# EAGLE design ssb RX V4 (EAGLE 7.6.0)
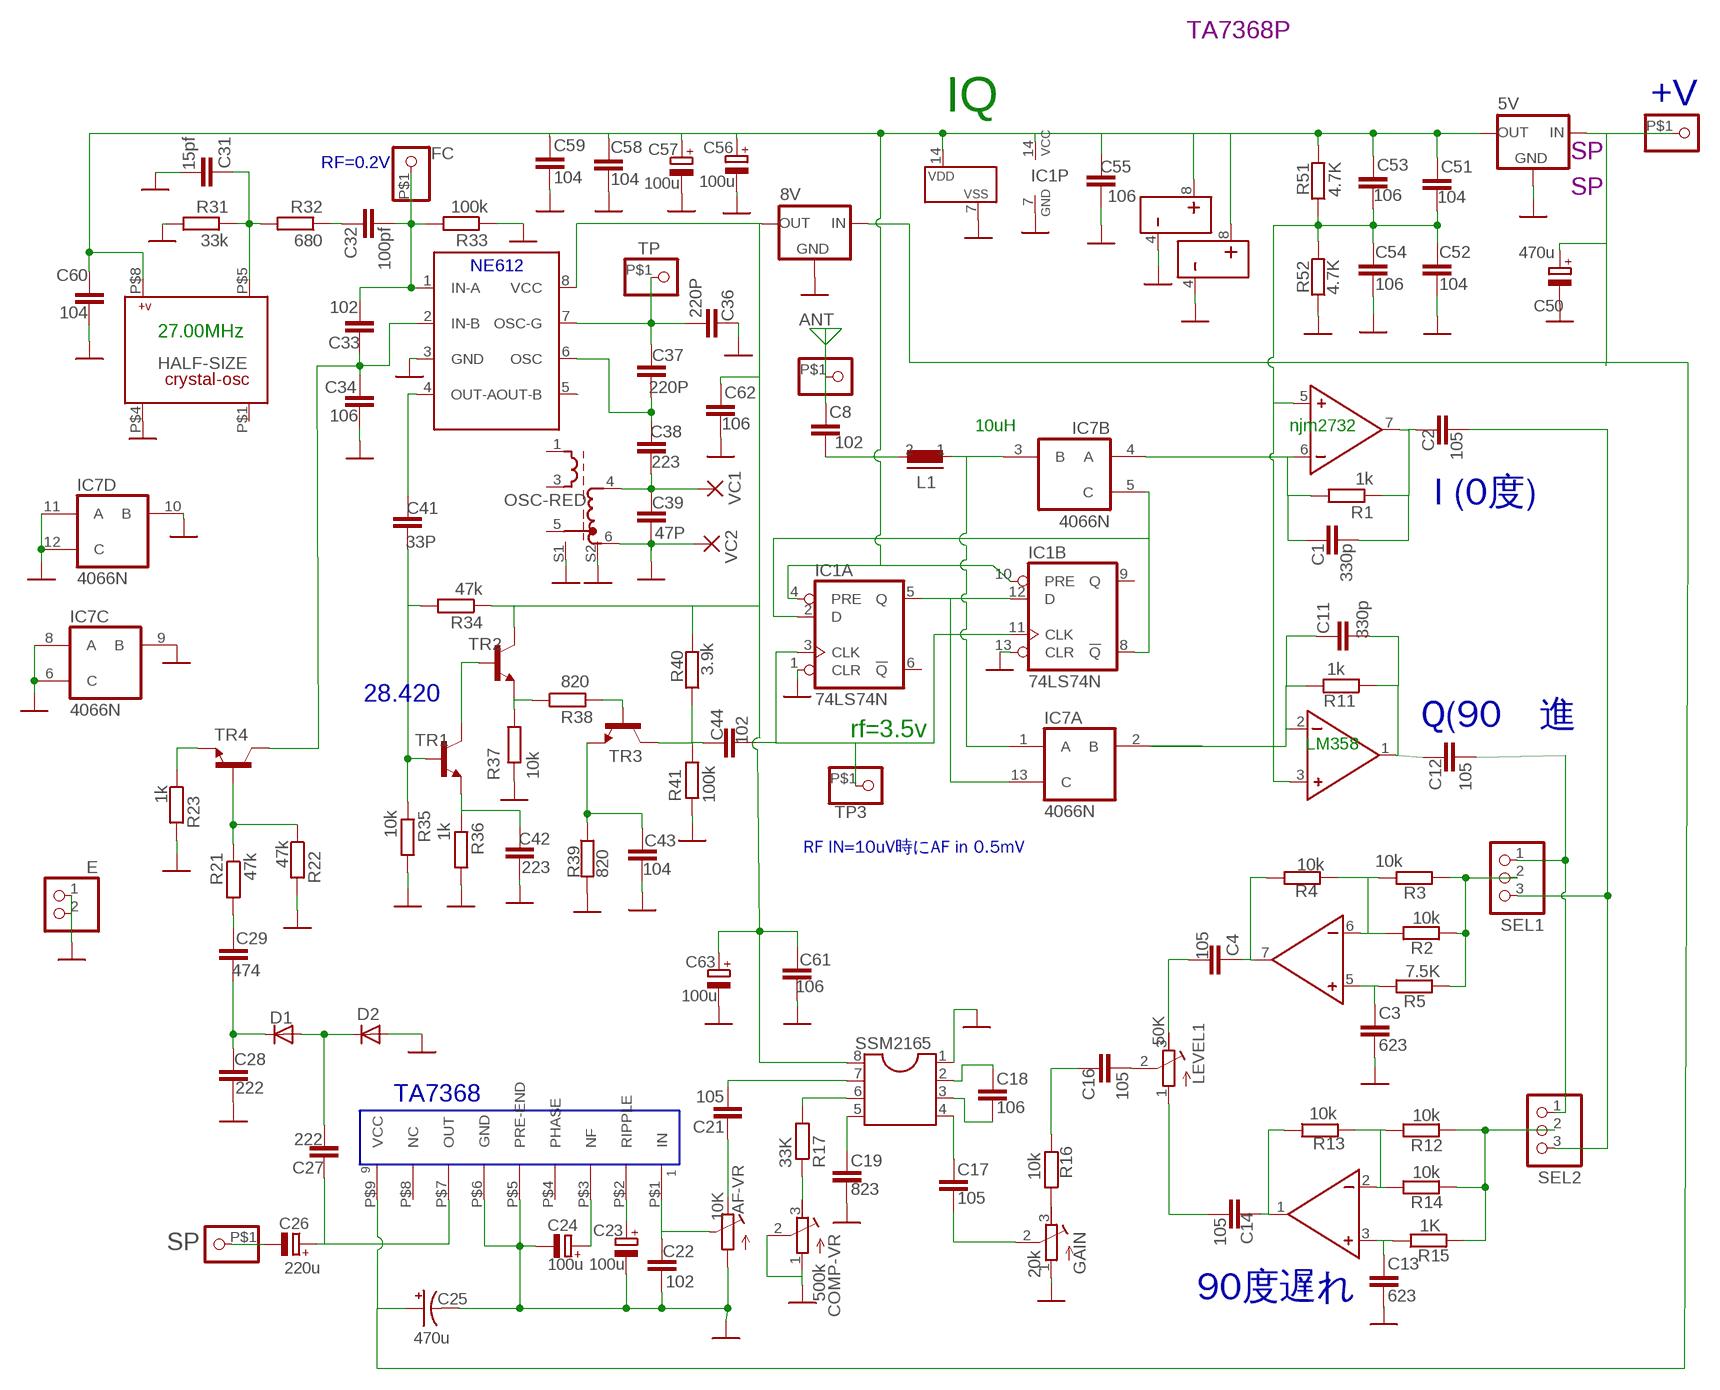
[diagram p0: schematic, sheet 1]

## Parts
5V  78MXX  [78MXX]
8V  78MXX  [78MXX]
+V  PINHD-1X1  [1X01]
AF-VR  10K  SINGLE-VR  [SINGLE-VR]
ANT  PINHD-1X1  [1X01]
C1  330p  C-EU050-024X044  [C050-024X044]
C2  105  C-EU050-024X044  [C050-024X044]
C3  623  C-EU050-024X044  [C050-024X044]
C4  105  C-EU050-024X044  [C050-024X044]
C8  102  C-EU050-024X044  [C050-024X044]
C11  330p  C-EU050-024X044  [C050-024X044]
C12  105  C-EU050-024X044  [C050-024X044]
C13  623  C-EU050-024X044  [C050-024X044]
C14  105  C-EU050-024X044  [C050-024X044]
C16  105  C-EU050-024X044  [C050-024X044]
C17  105  C-EU050-024X044  [C050-024X044]
C18  106  C-EU050-024X044  [C050-024X044]
C19  823  C-EU050-024X044  [C050-024X044]
C21  105  C-EU050-024X044  [C050-024X044]
C22  102  C-EU050-024X044  [C050-024X044]
C23  100u  CPOL-EUE2.5-6  [E2,5-6]
C24  100u  CPOL-EUE2.5-6  [E2,5-6]
C25  470u  CPOL-USE3.5-8  [E3,5-8]
C26  220u  CPOL-EUE2.5-6  [E2,5-6]
C27  222  C-EU050-024X044  [C050-024X044]
C28  222  C-EU050-024X044  [C050-024X044]
C29  474  C-EU050-024X044  [C050-024X044]
C31  15pf  C-EU050-024X044  [C050-024X044]
C32  100pf  C-EU050-024X044  [C050-024X044]
C33  102  C-EU050-024X044  [C050-024X044]
C34  106  C-EU050-024X044  [C050-024X044]
C36  220P  C-EU050-024X044  [C050-024X044]
C37  220P  C-EU050-024X044  [C050-024X044]
C38  223  C-EU050-024X044  [C050-024X044]
C39  47P  C-EU050-024X044  [C050-024X044]
C41  33P  C-EU050-024X044  [C050-024X044]
C42  223  C-EU050-024X044  [C050-024X044]
C43  104  C-EU050-024X044  [C050-024X044]
C44  102  C-EU050-024X044  [C050-024X044]
C50  470u  CPOL-EUE2.5-7  [E2,5-7]
C51  104  C-EU050-024X044  [C050-024X044]
C52  104  C-EU050-024X044  [C050-024X044]
C53  106  C-EU050-024X044  [C050-024X044]
C54  106  C-EU050-024X044  [C050-024X044]
C55  106  C-EU050-024X044  [C050-024X044]
C56  100u  CPOL-EUE2.5-6  [E2,5-6]
C57  100u  CPOL-EUE2.5-6  [E2,5-6]
C58  104  C-EU050-024X044  [C050-024X044]
C59  104  C-EU050-024X044  [C050-024X044]
C60  104  C-EU050-024X044  [C050-024X044]
C61  106  C-EU050-024X044  [C050-024X044]
C62  106  C-EU050-024X044  [C050-024X044]
C63  100u  CPOL-EUE2.5-6  [E2,5-6]
COMP-VR  500k  R-TRIMM3296W  [RTRIM3296W]
D1  DIODE-D-5  [D-5]
D2  DIODE-D-5  [D-5]
E  PINHD-1X2  [1X02]
FC  FC  PINHD-1X1  [1X01]
GAIN  20k  R-TRIMM3296W  [RTRIM3296W]
HALF-SIZE  X-OSC  [X-OSC]
IC1  74LS74N  [DIL14]
IC3  NE612  [NE612]
IC4  4558  [DIL08]
IC5  4558  [DIL08]
IC7  4066N  [DIL14]
JP1  SEL1  PINHD-1X3  [1X03]
JP3  SEL2  PINHD-1X3  [1X03]
L1  MCC10  [MCC10]
LEVEL1  50K  R-TRIMM3296W  [RTRIM3296W]
R1  1k  R-EU_0204/5  [0204/5]
R2  10k  R-EU_0204/5  [0204/5]
R3  10k  R-EU_0204/5  [0204/5]
R4  10k  R-EU_0204/5  [0204/5]
R5  7.5K  R-EU_0204/5  [0204/5]
R11  1k  R-EU_0204/5  [0204/5]
R12  10k  R-EU_0204/7  [0204/7]
R13  10k  R-EU_0204/5  [0204/5]
R14  10k  R-EU_0204/7  [0204/7]
R15  1K  R-EU_0204/5  [0204/5]
R16  10k  R-EU_0204/5  [0204/5]
R17  33K  R-EU_0204/5  [0204/5]
R21  47k  R-EU_0204/5  [0204/5]
R22  47k  R-EU_0204/5  [0204/5]
R23  1k  R-EU_0204/5  [0204/5]
R31  33k  R-EU_0204/5  [0204/5]
R32  680  R-EU_0204/5  [0204/5]
R33  100k  R-EU_0204/5  [0204/5]
R34  47k  R-EU_0204/5  [0204/5]
R35  10k  R-EU_0204/5  [0204/5]
R36  1k  R-EU_0204/5  [0204/5]
R37  10k  R-EU_0204/7  [0204/7]
R38  820  R-EU_0204/5  [0204/5]
R39  820  R-EU_0204/5  [0204/5]
R40  3.9k  R-EU_0204/5  [0204/5]
R41  100k  R-EU_0204/5  [0204/5]
R51  4.7K  R-EU_0204/5  [0204/5]
R52  4.7K  R-EU_0204/5  [0204/5]
SP  PINHD-1X1  [1X01]
SSM2165  LM386  [DIL08]
TA7368  TA7368P  [TA7368P]
TP  PINHD-1X1  [1X01]
TP3  PINHD-1X1  [1X01]
TR1  2SC1815L  [TO92-1815]
TR2  2SC1815L  [TO92-1815]
TR3  2SC1815L  [TO92-1815]
TR4  2SC1815L  [TO92-1815]
U$3  OSC-RED  [OSC-RED]
VC1  1,6/0,8  [1,6/0,8]
VC2  1,6/0,8  [1,6/0,8]

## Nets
9V: 5V.IN 8V.IN +V.P$1 C25.+ C50.+ TA7368.P$9(VCC)
GND: 5V.GND 8V.GND AF-VR.P$3(E) C3.2 C13.2 C19.2 C22.2 C23.- C24.- C25.- C28.2 C31.2 C34.2 C36.1 C39.2 C42.2 C43.1 C50.- C52.2 C54.2 C55.2 C56.- C57.- C58.2 C59.2 C60.2 C61.2 C62.2 C63.- COMP-VR.1(E) COMP-VR.2(S) D2.A E.1 E.2 GAIN.1(E) HALF-SIZE.P$4 IC1.1(A:CLR) IC1.7(P:GND) IC1.13(B:CLR) IC3.3(GND) IC4.4 IC5.4 IC7.6(C) IC7.7(VSS) IC7.8(A) IC7.9(B) IC7.10(B) IC7.11(A) IC7.12(C) R22.2 R23.2 R31.2 R33.1 R35.2 R36.2 R37.2 R39.2 R41.2 R52.1 SSM2165.1 TA7368.P$5(PRE-END) TA7368.P$6(GND) U$3.6 U$3.S1 U$3.S2 VC2.1(P)
N$2: IC5.6 R2.1 R3.1 R4.2
N$3: IC5.2 R12.1 R13.2 R14.1
N$4: AF-VR.P$1(A) C21.2
N$5: C4.2 IC5.7 R4.1
N$6: C3.1 IC5.5 R5.1
N$7: C12.1 JP1.1 JP3.1
N$8: C14.2 IC5.1 R13.1
N$9: C13.1 IC5.3 R15.1
N$10: C4.1 LEVEL1.3(A)
N$11: C32.1 R32.1
N$12: C16.1 LEVEL1.2(S)
N$13: GAIN.3(A) R16.1
N$14: C44.2 IC1.3(A:CLK) IC1.11(B:CLK) TP3.P$1
N$15: C11.1 C12.2 IC4.1 R11.1
N$16: IC1.5(A:Q) IC1.12(B:D) IC7.13(C)
N$17: JP3.2 R12.2 R14.2 R15.2
N$18: IC1.2(A:D) IC1.8(B:!Q) IC7.5(C)
N$19: C11.2 IC4.2 IC7.2(B) R11.2
N$20: IC7.1(A) IC7.3(B) L1.1
N$21: C1.1 C2.2 IC4.7 R1.1
N$22: C42.1 R36.1 TR1.E
N$23: C2.1 JP1.3 JP3.3
N$25: C1.2 IC4.6 IC7.4(A) R1.2
N$26: C14.1 LEVEL1.1(E)
N$27: 5V.OUT C51.1 C53.1 C55.1 C56.+ C57.+ C58.1 C59.1 C60.1 HALF-SIZE.P$8 IC1.4(A:PRE) IC1.10(B:PRE) IC1.14(P:VCC) IC4.8 IC5.8 IC7.14(VDD) R51.2
N$28: JP1.2 R2.2 R3.2 R5.2
N$29: C8.2 L1.2
N$30: ANT.P$1 C8.1
N$31: IC3.5(OUT-B)
N$32: AF-VR.P$2(S) C22.1 TA7368.P$1(IN)
N$33: C26.- SP.P$1
N$34: C51.2 C52.1 C53.2 C54.1 IC4.3 IC4.5 R51.1 R52.2
N$35: C32.2 C33.1 FC.P$1 IC3.1(IN-A) R33.2
N$36: C41.1 IC3.4(OUT-A)
N$39: C37.2 C38.1 IC3.6(OSC)
N$40: C36.2 C37.1 IC3.7(OSC-G) TP.P$1
N$41: C38.2 C39.1 U$3.4 VC1.1(P)
N$42: C41.2 R34.2 R35.1 TR1.B
N$43: R37.1 R38.1 TR2.E
N$44: C33.2 C34.1 IC3.2(IN-B) TR4.C
N$45: C17.1 SSM2165.4
N$46: TR1.C TR2.B
N$47: C31.1 HALF-SIZE.P$5 R31.1 R32.2
N$48: C26.+ C27.1 TA7368.P$7(OUT)
N$49: C24.+ TA7368.P$3(NF)
N$50: C23.+ TA7368.P$2(RIPPLE)
N$54: C21.1 SSM2165.7
N$57: C16.2 R16.2
N$58: C27.2 D1.A D2.C
N$59: C18.1 SSM2165.2
N$60: C18.2 SSM2165.3
N$62: C19.1 SSM2165.5
N$63: R17.2 SSM2165.6
N$64: COMP-VR.3(A) R17.1
N$65: C17.2 GAIN.2(S)
N$68: R23.1 TR4.E
N$71: R21.1 R22.1 TR4.B
N$73: C29.2 R21.2
N$74: C28.1 C29.1 D1.C
N$79: R38.2 TR3.B
N$80: C44.1 R40.1 R41.1 TR3.C
N$81: C43.2 R39.1 TR3.E
N$82: 8V.OUT C61.1 C62.1 C63.+ IC3.8(VCC) R34.1 R40.2 SSM2165.8 TR2.C
Unconnected: HALF-SIZE.P$1 IC1.6(A:!Q) IC1.9(B:Q) TA7368.P$4(PHASE) TA7368.P$8(NC) U$3.1 U$3.3 U$3.5

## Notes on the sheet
- TA7368P
- IQ
- SP
- RF=0.2V
- SP
- 27.00MHz
- 10uH | njm2732
- I (0度)
- 28.420
- Q(90　進
- rf=3.5v
- LM358
- RF IN=10uV時にAF in 0.5mV
- 90度遅れ

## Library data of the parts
5V 8V = v-reg:78MXX
+V ANT FC SP TP TP3 = pinhead:PINHD-1X1: PIN HEADER
AF-VR = resistor:SINGLE-VR
C1-C4 C8 C11-C14 C16-C19 C21 C22 C27-C29 C31-C34 C36-C39 C41-C44 C51-C55 C58-C62 = resistor:C-EU: CAPACITOR, European symbol
C23 C24 C26 C50 C56 C57 C63 = resistor:CPOL-EU: POLARIZED CAPACITOR, European symbol
C25 = resistor:CPOL-US: POLARIZED CAPACITOR, American symbol
COMP-VR GAIN LEVEL1 = resistor:R-TRIMM: Trimm resistor
D1 D2 = diode:DIODE-: DIODE
E = pinhead:PINHD-1X2: PIN HEADER
HALF-SIZE = OSC:X-OSC
IC1 = 74xx-us:74*74: Dual D type positive edge triggered FLIP FLOP, preset and clear
IC3 = ssm2166 :NE612
IC4 IC5 = ic-package:4558
IC7 = 40xx:4066: Quad bilateral ANALOG SWITCH
JP1 JP3 = pinhead:PINHD-1X3: PIN HEADER
L1 = inductors:MCC10: INDUCTOR
R1-R5 R11-R17 R21-R23 R31-R41 R51 R52 = resistor:R-EU_: RESISTOR, European symbol
SSM2165 = ic-package:LM386
TA7368 = lc7265:TA7368P
TR1-TR4 = transistor:2SC1815L
U$3 = OSC:OSC-RED
VC1 VC2 = wirepad:1,6/0,8: THROUGH-HOLE PAD

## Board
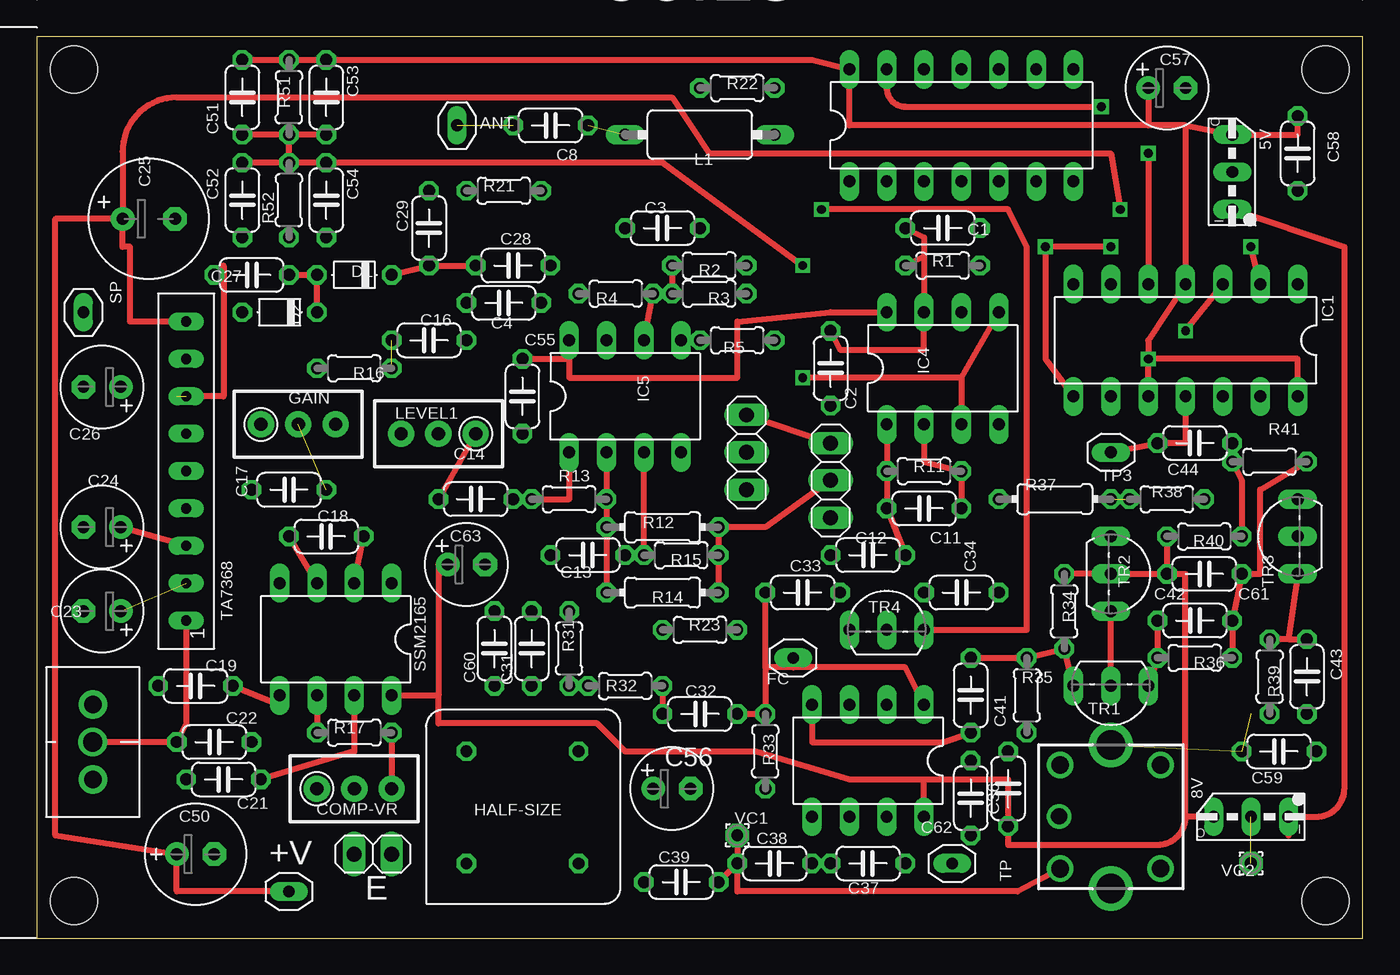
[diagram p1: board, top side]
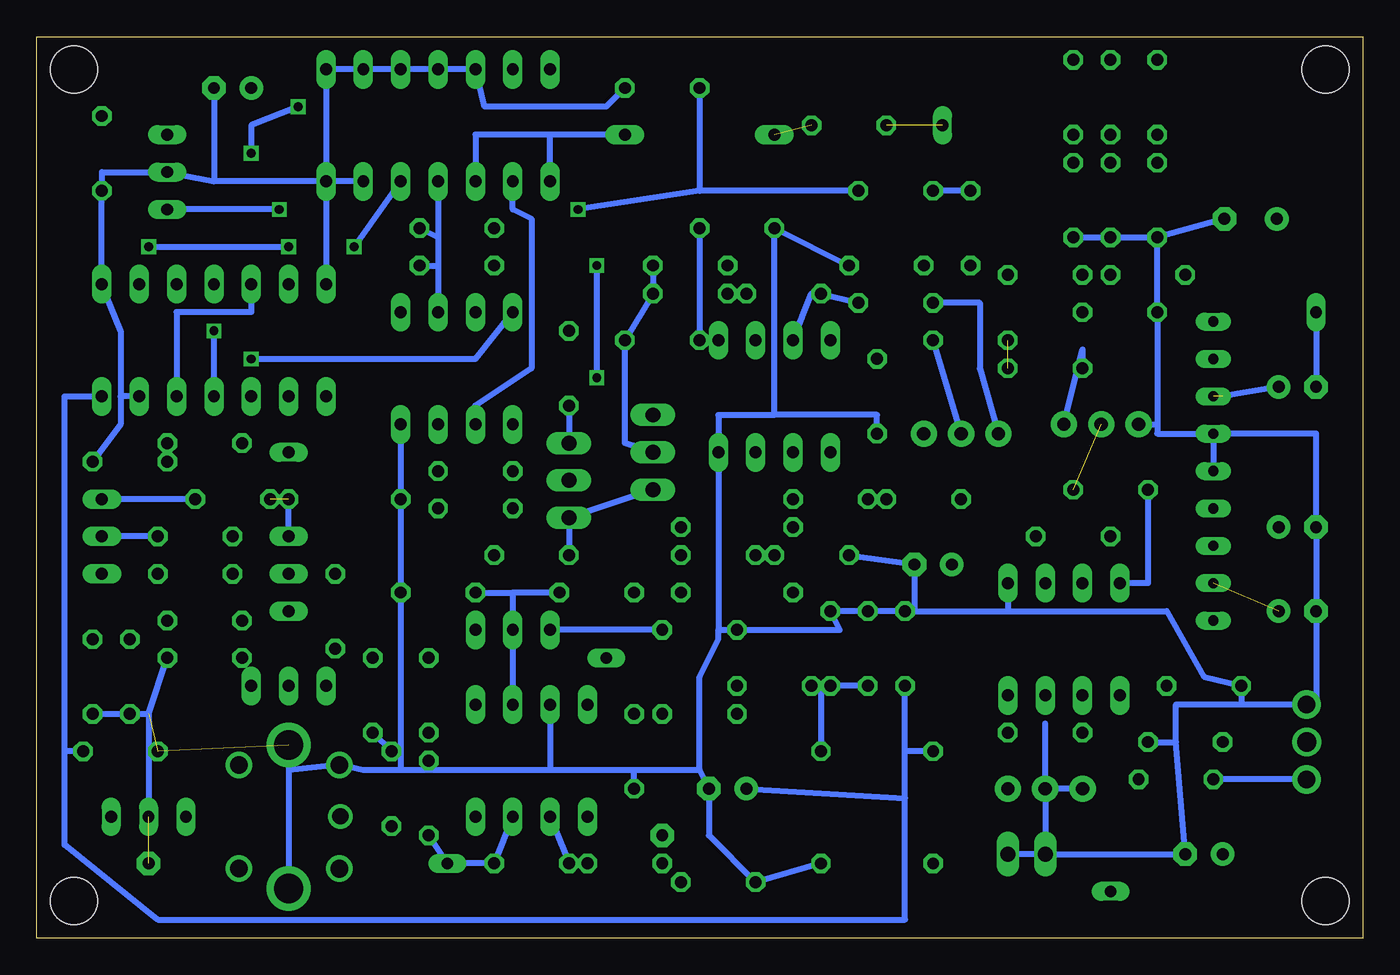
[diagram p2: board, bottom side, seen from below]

Size 90.15 x 61.27 mm. Coordinates in mm from the lower left corner, seen from the top.
Outline: 0,0 90.15,0 90.15,61.27 0,61.27 0,0
Copper layers (1*16): Top 0.035mm / dielectric 1.5mm / Bottom 0.035mm
Design rules "default": minimum track width 10mil, minimum drill 24mil, track to track 8mil, track to pad 8mil, pad to pad 8mil, via to via 8mil, smd to smd 8mil, copper to edge 40mil, drill to drill 8mil, minimum pad ring 10mil, minimum via ring 8mil, stop-mask expansion 4mil, vias tented up to drill 0mil, thermal gap 10mil
Holes 3.2 mm at 87.63,2.54 87.63,59.06 2.54,2.54 2.54,59.06

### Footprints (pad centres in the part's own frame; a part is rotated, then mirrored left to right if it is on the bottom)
78MXX = drill 0.8 pad 1.016 long: GND -2.54,1.27; IN -5.08,1.27; OUT 0,1.27
1X01 = drill 0.8 long: P$1 0,0
SINGLE-VR = drill 1.2 pad 1.93: P$1 0.635,2.54; P$3 0.635,-2.54 | drill 1.3 pad 1.93: P$2 0.635,0
C050-024X044 = drill 0.813 octagon: 1 -2.54,0; 2 2.54,0
E2,5-6 = drill 0.813 pad 1.6: + -1.27,0 | drill 0.813 pad 1.6 octagon: - 1.27,0
E3,5-8 = drill 0.813 pad 1.6: + -1.778,0 | drill 0.813 pad 1.6 octagon: - 1.778,0
E2,5-7 = drill 0.813 pad 1.6: + -1.27,0 | drill 0.813 pad 1.6 octagon: - 1.27,0
RTRIM3296W = drill 0.9 pad 1.778: 1 0,-2.54; 2 0,0; 3 0,2.54
D-5 = drill 0.813 octagon: A 2.54,0; C -2.54,0
1X02 = drill 1.016 long: 1 -1.27,0; 2 1.27,0
X-OSC = drill 0.8 octagon: P$1 -3.81,-3.81; P$4 3.81,-3.81; P$5 3.81,3.81; P$8 -3.81,3.81
DIL14 = drill 0.813 long: 1 -7.62,-3.81; 2 -5.08,-3.81; 3 -2.54,-3.81; 4 0,-3.81; 5 2.54,-3.81; 6 5.08,-3.81; 7 7.62,-3.81; 8 7.62,3.81; 9 5.08,3.81; 10 2.54,3.81; 11 0,3.81; 12 -2.54,3.81; 13 -5.08,3.81; 14 -7.62,3.81
NE612 = drill 0.813 long: 1 1.27,-3.81; 2 3.81,-3.81; 3 6.35,-3.81; 4 8.89,-3.81; 5 8.89,3.81; 6 6.35,3.81; 7 3.81,3.81; 8 1.27,3.81
DIL08 = drill 0.813 long: 1 -3.81,-3.81; 2 -1.27,-3.81; 3 1.27,-3.81; 4 3.81,-3.81; 5 3.81,3.81; 6 1.27,3.81; 7 -1.27,3.81; 8 -3.81,3.81
1X03 = drill 1.016 long: 1 -2.54,0; 2 0,0; 3 2.54,0
MCC10 = drill 0.813 long: 1 -5.08,0; 2 5.08,0
0204/5 = drill 0.813 octagon: 1 -2.54,0; 2 2.54,0
0204/7 = drill 0.813 octagon: 1 -3.81,0; 2 3.81,0
TA7368P = drill 0.7 long: P$1 -6.35,1.27; P$2 -3.81,1.27; P$3 -1.27,1.27; P$4 1.27,1.27; P$5 3.81,1.27; P$6 6.35,1.27; P$7 8.89,1.27; P$8 11.43,1.27; P$9 13.97,1.27
TO92-1815 = drill 0.813 long: B 2.54,0; C 0,0; E -2.54,0
OSC-RED = drill 1.2: 1 -3.39,3.518; 3 -3.39,-3.518; 4 3.454,3.531; 6 3.454,-3.518 | drill 1.1: 5 3.518,-0.025 | drill 2: S1 0,-4.873; S2 0,4.873
1,6/0,8 = drill 0.813 pad 1.6 octagon: 1 0,0

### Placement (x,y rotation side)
5V  82.55,54.61 90 top
8V  80.01,9.52 180 top
+V  17.15,3.18 0 top
AF-VR  4.45,13.34 180 top
ANT  28.58,55.25 90 top
C1  61.59,48.26 0 top
C2  53.97,38.73 90 top
C3  42.55,48.26 180 top
C4  31.75,43.18 0 top
C8  34.92,55.25 0 top
C11  60.33,29.21 0 top
C12  56.52,26.03 0 top
C13  37.47,26.03 180 top
C14  29.84,29.84 0 top
C16  26.67,40.64 180 top
C17  17.15,30.48 0 top
C18  19.69,27.3 180 top
C19  10.8,17.15 180 top
C21  12.7,10.8 180 top
C22  12.06,13.34 0 top
C23  4.45,22.23 180 top
C24  4.45,27.94 180 top
C25  7.62,48.89 0 top
C26  4.45,37.47 180 top
C27  14.6,45.09 0 top
C28  32.39,45.72 0 top
C29  26.67,48.26 90 top
C31  33.66,19.69 90 top
C32  45.08,15.24 0 top
C33  52.07,23.49 0 top
C34  62.86,23.49 0 top
C36  63.5,9.52 270 top
C37  56.52,5.08 180 top
C38  50.17,5.08 180 top
C39  43.81,3.81 180 top
C41  63.5,16.51 90 top
C42  78.74,21.59 0 top
C43  86.36,17.78 90 top
C44  78.74,33.66 180 top
C50  10.8,5.71 0 top
C51  13.97,57.15 270 top
C52  13.97,50.17 270 top
C53  19.69,57.15 270 top
C54  19.69,50.17 270 top
C55  33.02,36.83 270 top
C56  43.18,10.16 0 top
C57  76.83,57.78 0 top
C58  85.72,53.34 270 top
C59  84.45,12.7 180 top
C60  31.12,19.69 90 top
C61  79.38,24.77 0 top
C62  66.04,10.16 90 top
C63  29.21,25.4 0 top
COMP-VR  21.59,10.16 270 top
D1  21.59,45.09 180 top
D2  16.51,42.55 180 top
E  22.86,5.71 180 top
FC  51.44,19.05 180 top
GAIN  17.78,34.92 270 top
HALF-SIZE  33.02,8.89 0 top
IC1  78.11,40.64 180 top
IC3  61.59,12.07 180 top
IC4  61.59,38.73 0 top
IC5  40,36.83 0 top
IC7  62.86,55.25 0 top
JP1  48.26,33.02 90 top
JP3  53.97,31.12 90 top
L1  45.08,54.61 180 top
LEVEL1  27.3,34.29 90 top
R1  61.59,45.72 0 top
R2  45.72,45.72 0 top
R3  45.72,43.81 0 top
R4  39.37,43.81 0 top
R5  47.62,40.64 0 top
R11  60.33,31.75 0 top
R12  42.55,27.94 0 top
R13  36.19,29.84 0 top
R14  42.55,23.49 0 top
R15  43.81,26.03 0 top
R16  21.59,38.73 0 top
R17  21.59,13.97 180 top
R21  31.75,50.8 180 top
R22  47.62,57.78 0 top
R23  45.08,20.95 180 top
R31  36.19,19.69 90 top
R32  40,17.15 180 top
R33  49.53,12.7 90 top
R34  69.85,22.23 270 top
R35  67.31,16.51 270 top
R36  78.74,19.05 0 top
R37  69.22,29.84 180 top
R38  76.83,29.84 0 top
R39  83.82,17.78 270 top
R40  79.38,27.3 180 top
R41  83.82,32.38 0 top
R51  17.15,57.15 90 top
R52  17.15,50.17 90 top
SP  3.17,42.55 90 top
SSM2165  20.32,20.32 180 top
TA7368  11.43,27.94 90 top
TP  62.23,5.08 180 top
TP3  73.03,33.02 0 top
TR1  73.03,17.15 180 top
TR2  73.03,24.77 270 top
TR3  85.72,27.3 90 top
TR4  57.78,20.95 0 top
U$3  73.03,8.25 180 top
VC1  47.62,6.98 0 top
VC2  82.55,5.08 0 top

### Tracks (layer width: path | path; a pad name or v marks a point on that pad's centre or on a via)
9V  (via drill 0.6)
  Top 0.406: 5V.IN 88.9,46.99 88.9,10.16 arc-90 87,8.25 8V.IN 85.09,6.98 | v73.66,49.53 73.03,53.34 45.72,53.34 43.18,57.15 9.52,57.15 arc90 5.84,53.47 C25.+ | C25.+ 1.27,48.89 1.27,6.98 C50.+ 9.52,3.18 +V.P$1 | TA7368.P$9 6.35,41.91 6.35,46.99 5.84,46.99 C25.+
  Bottom 0.406: v73.66,49.53 5V.IN
GND  (3 unrouted)
  Top 0.406: R41.2 83.19,30.48 83.19,24.77 C61.2 C42.2 R36.2
  Bottom 0.406: IC7.7 IC1.7 | IC7.6 IC7.7 | IC7.7 IC7.8 IC7.9 IC7.10 IC7.11 IC7.12 59.69,56.52 51.44,56.52 R22.2 | TA7368.P$6 TA7368.P$5 | 55.25,11.43 IC3.3 55.25,16.51 | 84.45,36.83 84.45,41.27 IC1.1 C58.2 85.72,52.07 5V.GND 78.11,51.44 | 84.45,36.83 84.45,34.92 R41.2 | IC1.13 84.45,36.83 | IC7.7 78.11,51.44 | E.2 E.1 | C13.2 C63.- 30.48,22.23 | 82.55,15.24 R36.2 | 82.55,15.24 R39.2 C43.1 | 82.55,15.24 8V.GND | IC4.4 R37.2 C34.2 65.41,12.7 | U$3.S1 73.03,11.43 | 73.03,11.43 U$3.S2 | 30.48,22.23 C60.2 C31.2 R31.2 35.56,20.95 R23.2 43.81,20.95 | 43.81,20.95 IC5.4 43.81,35.56 40,35.56 | TA7368.P$6 3.17,34.29 C24.- C23.- 3.17,15.88 AF-VR.P$3 8.26,15.88 | 45.08,11.43 45.08,17.78 43.81,20.32 43.81,20.95 | 8.26,15.88 12.7,15.88 12.7,13.34 | 12.7,13.34 C50.- E.2 | C22.2 12.7,13.34 | SSM2165.1 24.13,22.23 | C54.2 R52.1 C52.2 | 13.97,34.92 D2.A C52.2 | 13.97,34.92 13.97,34.29 TA7368.P$6 | GAIN.1 13.97,34.92 | C28.2 C3.2 40,35.56 | C55.2 33.02,35.56 40,35.56 | C25.- C52.2 | 30.48,22.23 24.13,22.23 | COMP-VR.2 21.59,14.61 | COMP-VR.1 COMP-VR.2 | 8.26,15.88 C19.2 10.8,17.78 13.34,22.23 24.13,22.23 | COMP-VR.2 E.2 | HALF-SIZE.P$4 C39.2 44.45,6.98 C56.- 45.08,11.43 | 55.25,11.43 63.5,11.43 | 63.5,11.43 65.41,11.43 | C36.1 63.5,11.43 | R35.2 C62.2 65.41,12.7 | 65.41,11.43 67.94,11.43 U$3.6 73.03,11.43 | 65.41,12.7 65.41,11.43 | 45.08,11.43 49.53,11.43 | 49.53,11.43 55.25,11.43 | R33.1 49.53,11.43 | C57.- 78.11,51.44
N$2
  Top 0.406: IC5.6 R4.2 R3.1 R2.1
N$3
  Top 0.406: IC5.2 R13.2 R12.1 R14.1
N$4
  Bottom 0.406: AF-VR.P$1 C21.2
N$5
  Bottom 0.406: C4.2 R4.1 37.47,43.81 IC5.7
N$6
  Bottom 0.406: IC5.5 R5.1 C3.1
N$7
  Bottom 0.406: JP1.1 JP3.1 C12.1
N$8
  Top 0.406: IC5.1 36.19,29.84 R13.1 C14.2
N$9
  Top 0.406: C13.1 R15.1 IC5.3
N$10
  Bottom 0.406: C4.1 26.03,43.18 26.03,38.73 LEVEL1.3
N$11
  Top 0.406: R32.1 C32.1
N$12
  Bottom 0.406: C16.1 LEVEL1.2
N$13
  Bottom 0.406: GAIN.3 19.05,40.01 R16.1
N$14  (via drill 0.6)
  Top 0.406: IC1.11 78.11,33.66 C44.2 TP3.P$1 | v78.11,41.27 IC1.3
  Bottom 0.406: IC1.11 v78.11,41.27
N$15
  Top 0.406: IC4.1 R11.1 C11.1 C12.2
N$16  (via drill 0.6)
  Top 0.406: IC7.13 57.78,57.78 arc90 59.06,56.52 v72.39,56.52 | v75.56,53.34 IC1.5
  Bottom 0.406: IC1.5 75.56,42.55 80.64,42.55 IC1.12 | v72.39,56.52 75.56,55.25 v75.56,53.34
N$17
  Top 0.406: JP3.2 49.53,27.94 R12.2 R15.2 R14.2
N$18  (via drill 0.6)
  Top 0.406: IC1.8 68.58,39.37 v68.58,46.99 v73.03,46.99 | IC1.2 v82.55,46.99
  Bottom 0.406: IC7.5 v68.58,46.99 | v82.55,46.99 v73.03,46.99
N$19
  Top 0.406: C11.2 R11.2 60.33,32.38 IC4.2
  Bottom 0.406: IC7.2 57.78,49.53 56.52,48.89 56.52,38.73 60.33,36.2 IC4.2
N$20
  Bottom 0.406: IC7.1 55.25,54.61 | 55.25,54.61 60.33,54.61 IC7.3 | L1.1 55.25,54.61
N$21
  Top 0.406: C1.1 60.33,47.62 60.33,46.35 | 60.33,46.35 IC4.7 60.33,40.01 54.61,40.01 C2.2 | R1.1 60.33,46.35
N$22
  Top 0.406: C42.1 R36.1 TR1.E
N$23
  Top 0.406: JP1.3 JP3.3
  Bottom 0.406: C2.1 JP3.3
N$25
  Bottom 0.406: 62.86,47.62 62.86,45.72 | 62.86,45.72 IC4.6 | R1.2 62.86,45.72 | C1.2 62.86,47.62 | IC7.4 62.86,47.62
N$26
  Top 0.406: LEVEL1.1 C14.1
N$27  (via drill 0.6)
  Top 0.406: 78.11,55.25 IC1.4 75.56,40.64 v75.56,39.37 | 78.11,55.25 75.56,55.25 | 75.56,55.25 55.25,55.25 IC7.14 52.7,59.69 C53.1 R51.2 C51.1 | IC1.14 85.72,39.37 v75.56,39.37 | IC5.8 36.19,39.37 | 36.19,39.37 36.19,38.1 47.62,38.1 47.62,41.91 53.97,42.55 IC4.8 | 78.11,55.25 5V.OUT 85.72,54.61 C58.1 | C55.1 36.19,39.37 | IC1.10 v75.56,39.37 | C57.+ 75.56,55.25
  Bottom 0.406: 31.12,9.52 31.12,1.27 81.92,1.27 88.27,6.35 88.27,12.7 | 31.12,9.52 31.12,12.7 | HALF-SIZE.P$8 31.12,12.7 | 88.27,12.7 88.27,36.83 IC1.14 | C59.1 88.27,12.7 | 31.12,12.7 C60.1 | v75.56,39.37 60.33,39.37 IC4.8 | C56.+ 31.12,9.52
N$28
  Bottom 0.406: JP1.2 50.17,33.66 R5.2 R3.2 R2.2
N$29  (1 unrouted)
N$30  (1 unrouted)
N$32
  Top 0.406: AF-VR.P$2 C22.1 10.16,14.61 TA7368.P$1
N$33
  Bottom 0.406: SP.P$1 C26.-
N$34  (via drill 0.6)
  Top 0.406: 62.86,38.1 IC4.5 | 62.86,38.1 v52.07,38.1 | v52.07,45.72 42.55,52.7 C54.1 R52.2 | R51.1 C51.2 | 62.86,38.1 IC4.3 | R52.2 C52.1 | R52.2 R51.1 | C53.2 R51.1
  Bottom 0.406: v52.07,38.1 v52.07,45.72
N$35
  Top 0.406: IC3.1 59.06,18.41 51.44,18.41 | 51.44,18.41 49.53,18.41 | 49.53,18.41 C33.1 | 49.53,18.41 R33.2 C32.2 | FC.P$1 51.44,18.41
N$36
  Top 0.406: IC3.4 52.7,13.34 61.59,13.34 C41.1
N$39
  Bottom 0.406: C38.1 C37.2 IC3.6
N$40
  Bottom 0.406: IC3.7 C37.1 TP.P$1 C36.2
N$41
  Top 0.406: U$3.4 66.67,3.18 47.62,3.18 C38.2 | C38.2 C39.1 | VC1.1 C38.2
N$42
  Top 0.406: C41.2 R35.1 R34.2 TR1.B
N$43  (1 unrouted)
  Bottom 0.406: TR2.E R37.1
N$44
  Bottom 0.406: 57.78,23.49 TR4.C IC3.2 | C33.2 57.78,23.49 | C34.1 57.78,23.49
N$45
  Bottom 0.406: C17.1 14.6,24.13 SSM2165.4
N$46
  Top 0.406: TR1.C TR2.B
N$47
  Bottom 0.406: C31.1 R31.1 36.83,17.15 | 36.83,17.15 HALF-SIZE.P$5 | R32.2 36.83,17.15
N$48  (1 unrouted)
  Top 0.406: C27.1 12.7,45.72 12.7,36.83 TA7368.P$7
  Bottom 0.406: C26.+ 9.52,36.83
N$49
  Top 0.406: TA7368.P$3 C24.+
N$50  (1 unrouted)
N$54
  Top 0.406: SSM2165.7 21.59,12.7 C21.1
N$57  (1 unrouted)
N$58
  Top 0.406: C27.2 D1.A D2.C
N$59
  Top 0.406: SSM2165.2 C18.1
N$60
  Top 0.406: SSM2165.3 C18.2
N$62
  Top 0.406: C19.1 16.51,15.88 SSM2165.5
N$63
  Top 0.406: SSM2165.6 R17.2
N$64
  Top 0.406: R17.1 COMP-VR.3
N$65  (1 unrouted)
N$68
  Bottom 0.406: R23.1 TR4.E
N$71  (via drill 0.6)
  Top 0.406: TR4.B 67.31,20.95 67.31,46.99 66.04,49.53 v53.34,49.53
  Bottom 0.406: R22.1 45.08,50.8 | 45.08,50.8 v53.34,49.53 | R21.1 45.08,50.8
N$73
  Bottom 0.406: C29.2 R21.2
N$74
  Top 0.406: D1.C C29.1 C28.1
N$79
  Bottom 0.406: R38.2 TR3.B
N$80
  Top 0.406: C44.1 R41.1 81.92,31.12 R40.1
  Bottom 0.406: R40.1 TR3.C
N$81
  Top 0.406: TR3.E 85.09,20.32 | 85.09,20.32 R39.1 | 85.09,20.32 C43.2
N$82
  Top 0.406: R34.1 TR2.C C61.1 | 8V.OUT 78.11,8.25 | 78.11,8.25 78.11,24.77 C61.1 | R40.2 C61.1 | 60.33,10.8 55.25,10.8 48.89,12.7 40,12.7 38.1,14.61 27.3,14.61 27.3,16.51 | SSM2165.8 27.3,16.51 | C63.+ 27.3,25.4 27.3,16.51 | 78.11,8.25 arc-90 76.2,6.35 66.04,6.35 C62.1 66.04,10.8 60.33,10.8 | IC3.8 60.33,10.8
